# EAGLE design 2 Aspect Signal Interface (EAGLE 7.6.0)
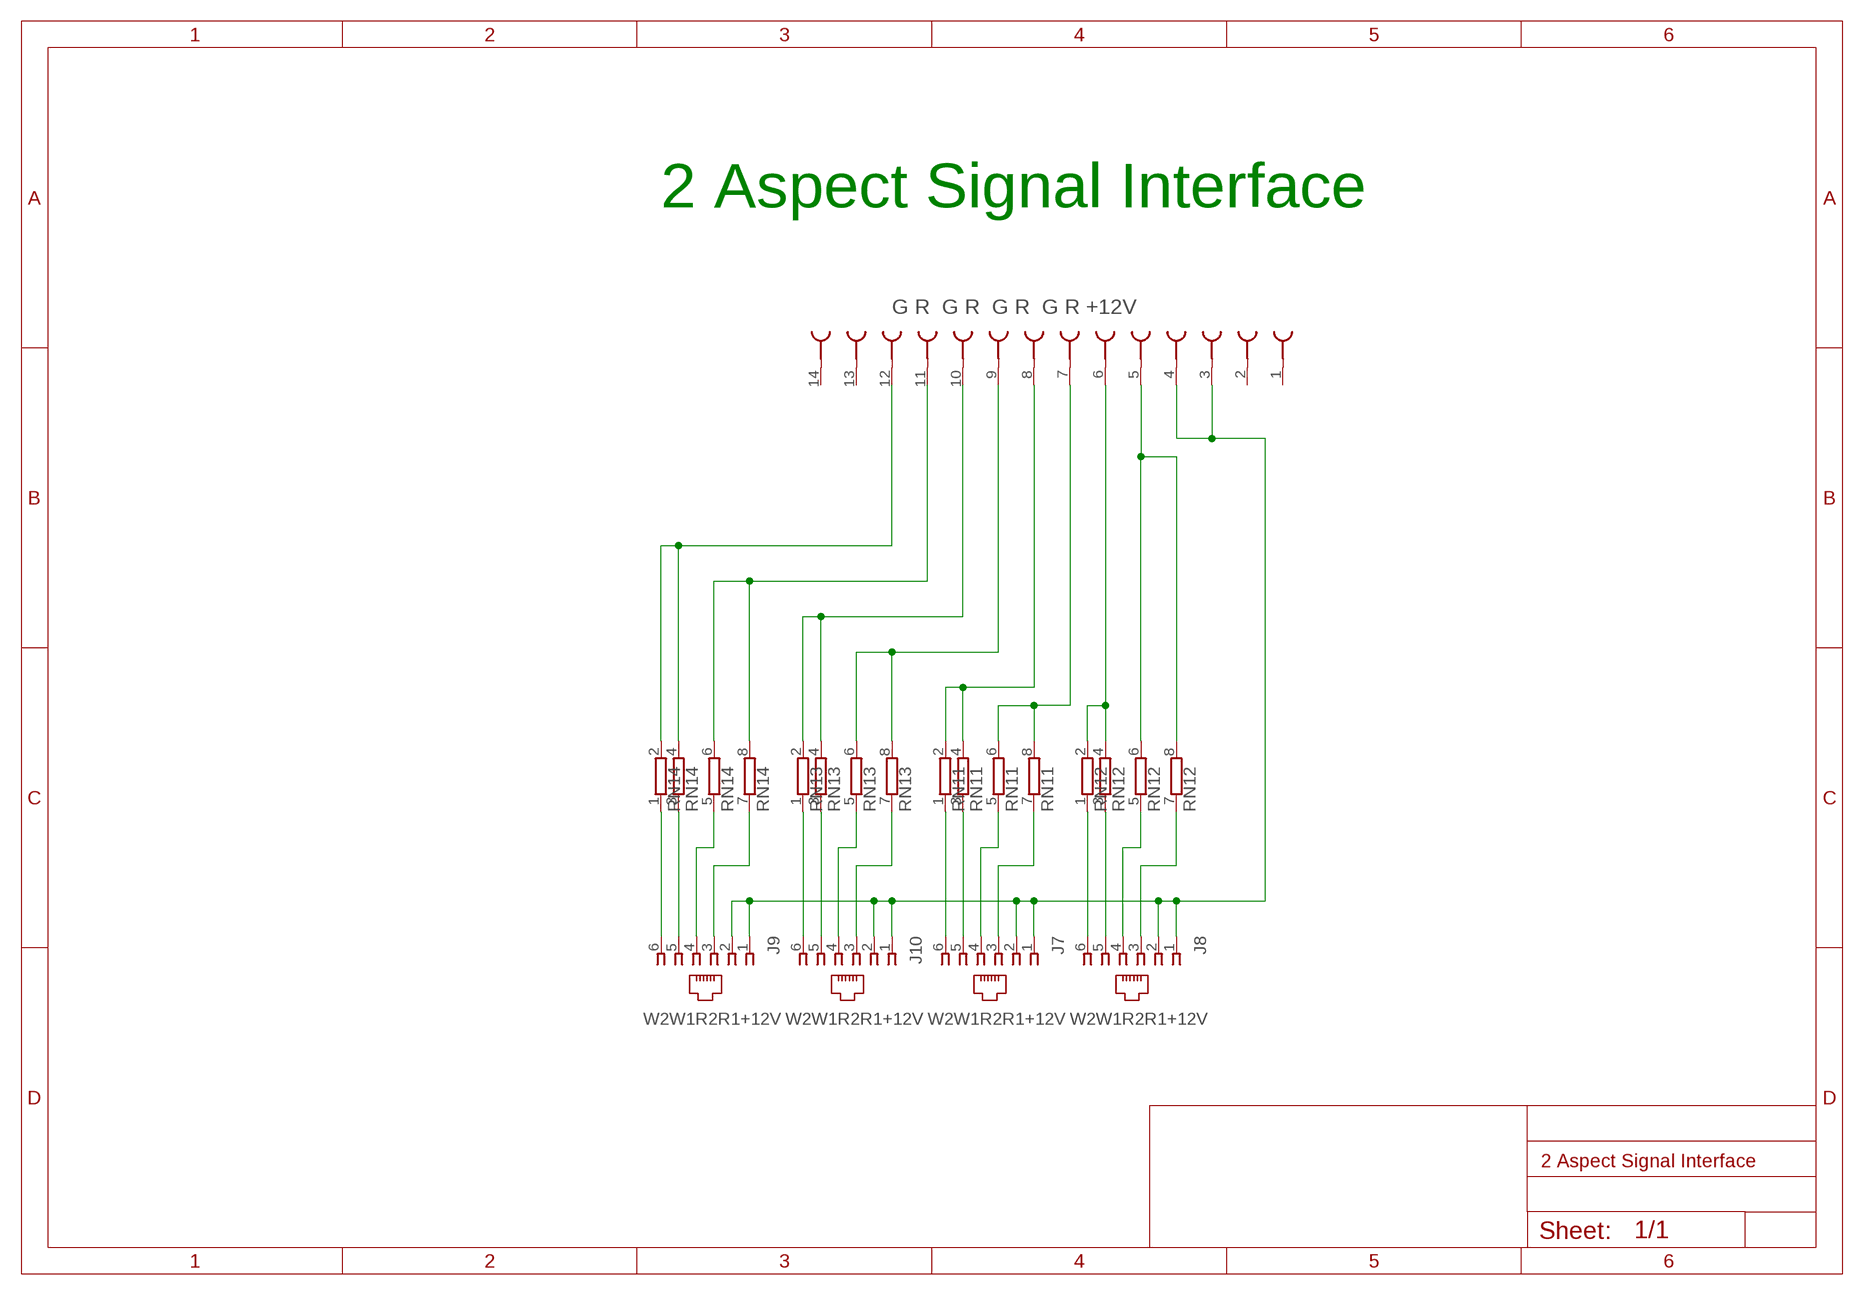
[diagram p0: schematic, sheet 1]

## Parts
J7  520250-3  [520250-3]
J8  520250-3  [520250-3]
J9  520250-3  [520250-3]
J10  520250-3  [520250-3]
RN11  E4RP  [SIL8]
RN12  E4RP  [SIL8]
RN13  E4RP  [SIL8]
RN14  E4RP  [SIL8]
U$16  AMP_FEMALE_PLUG  [AMP_FEMALE_PLUG]

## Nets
N$65: RN12.2 RN12.4 U$16.6(SK5)
N$66: J7.4 RN11.5
N$67: J7.5 RN11.3
N$68: J7.6 RN11.1
N$69: J7.3 RN11.7
N$70: J10.4 RN13.5
N$71: J8.5 RN12.3
N$72: J8.6 RN12.1
N$73: RN12.6 RN12.8 U$16.5(SK4)
N$74: J8.4 RN12.5
N$75: J10.3 RN13.7
N$76: RN11.6 RN11.8 U$16.7(SK6)
N$77: J8.3 RN12.7
N$78: J10.5 RN13.3
N$79: J10.6 RN13.1
N$80: J9.4 RN14.5
N$81: J9.3 RN14.7
N$85: J9.5 RN14.3
N$86: J9.6 RN14.1
N$87: J7.1 J7.2 J8.1 J8.2 J9.1 J9.2 J10.1 J10.2 U$16.3(SK2) U$16.4(SK3)
N$89: RN11.2 RN11.4 U$16.8(SK7)
N$90: RN13.6 RN13.8 U$16.9(SK8)
N$91: RN13.2 RN13.4 U$16.10(SK9)
N$92: RN14.6 RN14.8 U$16.11(SK10)
N$93: RN14.2 RN14.4 U$16.12(SK11)
Unconnected: U$16.1(SK) U$16.2(SK1) U$16.13(SK12) U$16.14(SK13)

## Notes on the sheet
- 2 Aspect Signal Interface
- G R  G R  G R  G R +12V
- W2W1R2R1+12V | W2W1R2R1+12V | W2W1R2R1+12V | W2W1R2R1+12V

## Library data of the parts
J7-J10 = con-amp:520250-3: AMP connector; MF: TYCO ELECTRONICS; MPN: 5520250-3; OC_FARNELL: unknown; OC_NEWARK: 42K8724
RN11-RN14 = resistor-sil:E4RP: SIL RESISTOR; OC_FARNELL: unknown; OC_NEWARK: unknown
U$16 = con-3m:AMP_FEMALE_PLUG

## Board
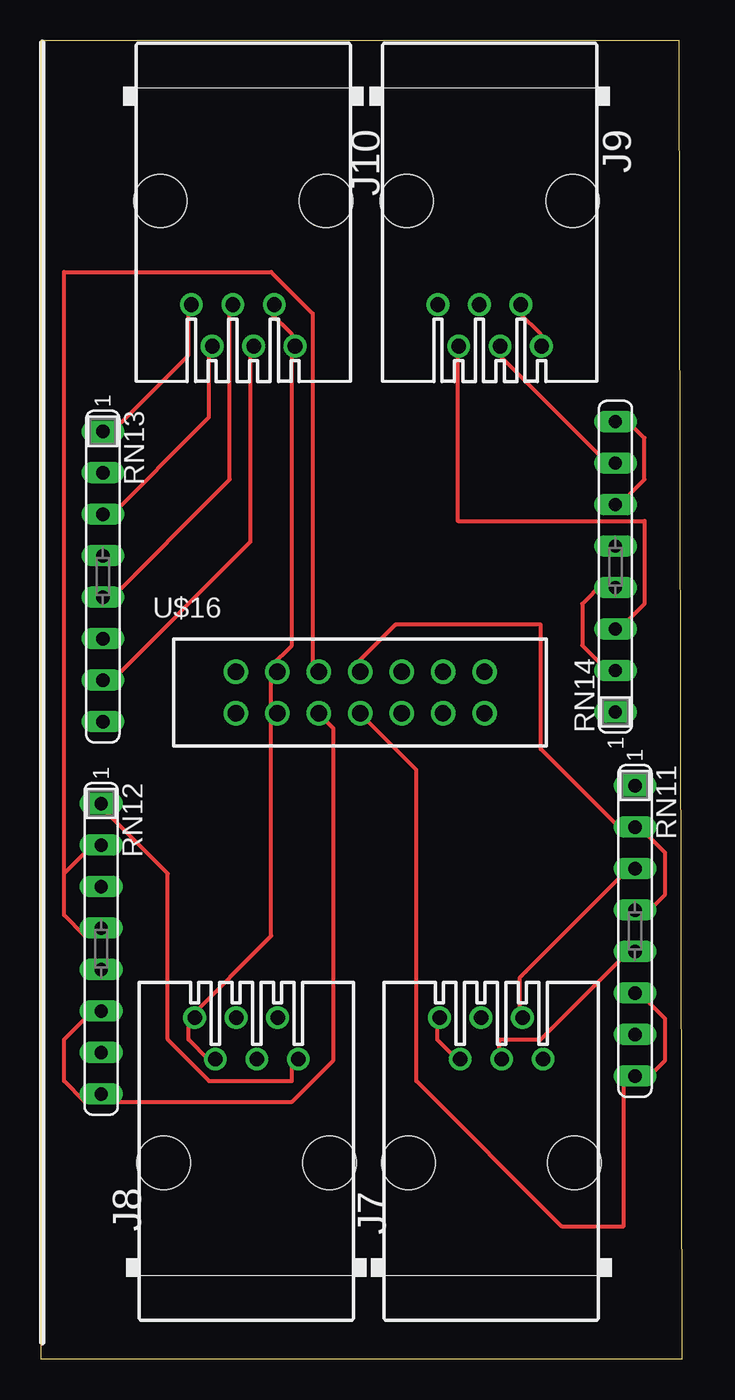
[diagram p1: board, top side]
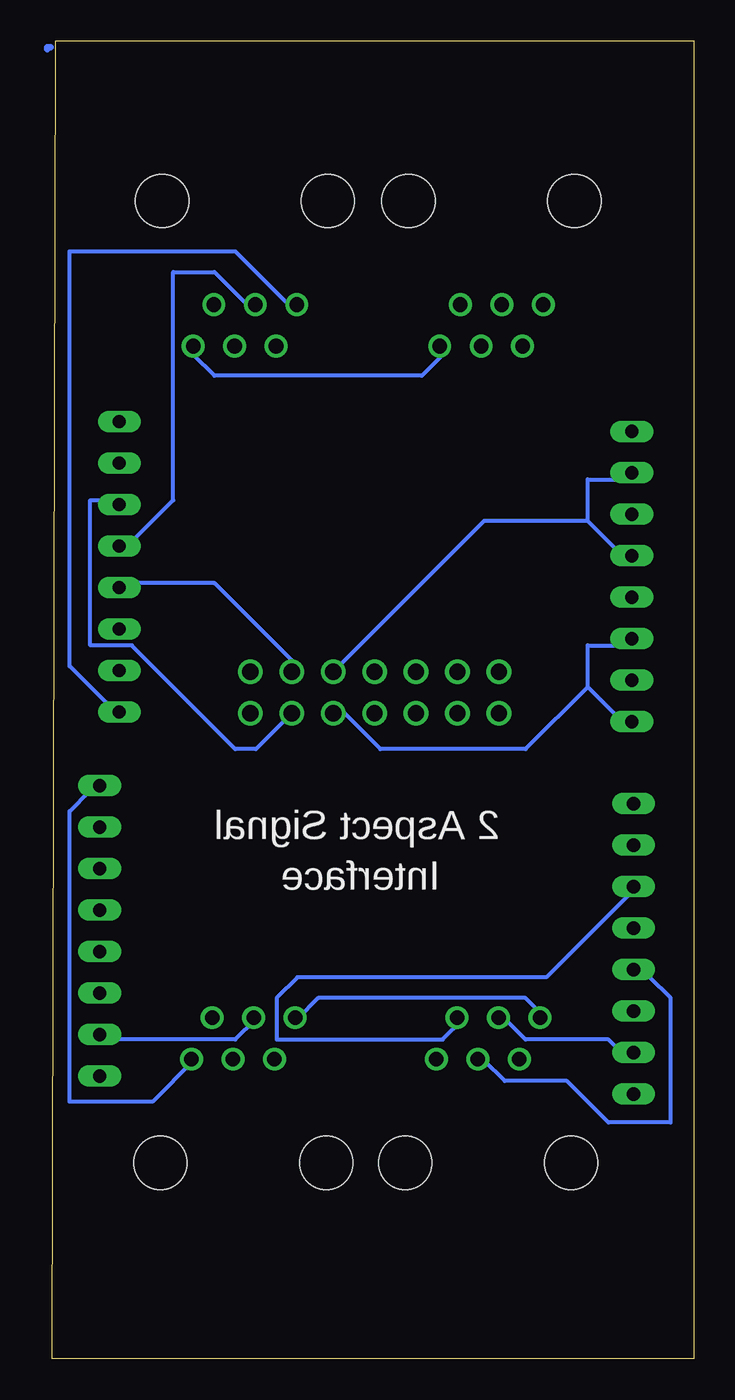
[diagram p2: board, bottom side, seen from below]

Size 39.3 x 80.7 mm. Coordinates in mm from the lower left corner, seen from the top.
Outline: 0,0 39.3,0 39.1,80.7 0,80.7 0,0
Copper layers (1*16): Top 0.035mm / dielectric 1.5mm / Bottom 0.035mm
Design rules "default": minimum track width 10mil, minimum drill 24mil, track to track 8mil, track to pad 8mil, pad to pad 8mil, via to via 8mil, smd to smd 8mil, copper to edge 40mil, drill to drill 8mil, minimum pad ring 10mil, minimum via ring 8mil, stop-mask expansion 4mil, vias tented up to drill 0mil, thermal gap 10mil

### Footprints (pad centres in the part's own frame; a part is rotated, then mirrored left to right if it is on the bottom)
520250-3 = drill 0.889: 1 -3.175,8.89; 2 -1.905,6.35; 3 -0.635,8.89; 4 0.635,6.35; 5 1.905,8.89; 6 3.175,6.35 | hole 3.251: -5.08,0; 5.08,0
SIL8 = drill 0.813 long: 1 -8.89,0; 2 -6.35,0; 3 -3.81,0; 4 -1.27,0; 5 1.27,0; 6 3.81,0; 7 6.35,0; 8 8.89,0
AMP_FEMALE_PLUG = drill 1 pad 1.422: 1 -10.16,-1.27; 2 -10.16,1.27; 3 -7.62,-1.27; 4 -7.62,1.27; 5 -5.08,-1.27; 6 -5.08,1.27; 7 -2.54,-1.27; 8 -2.54,1.27; 9 0,-1.27; 10 0,1.27; 11 2.54,-1.27; 12 2.54,1.27; 13 5.08,-1.27; 14 5.08,1.27

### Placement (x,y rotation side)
J7  27.6,12 0 top
J8  12.6,12 0 top
J9  27.5,70.9 180 top
J10  12.4,70.9 180 top
RN11  36.4,26.2 270 top
RN12  3.7,25.1 270 top
RN13  3.8,47.9 270 top
RN14  35.2,48.5 90 top
U$16  22.1,40.8 0 top

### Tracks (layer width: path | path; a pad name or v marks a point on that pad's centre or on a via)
N$65
  Top 0.254: 1.42,29.71 1.42,27.17 2.69,25.9 RN12.4 | 1.42,29.71 2.69,30.98 RN12.2 | 1.42,29.71 1.42,66.54 14.12,66.54 16.66,64 16.66,42.41 U$16.6
N$66
  Top 0.254: RN11.5 35.71,24.63 30.63,19.55 28.09,19.55 28.09,18.28 J7.4
N$67
  Top 0.254: RN11.3 35.71,29.71 29.36,23.36 29.36,20.82 J7.5
N$68
  Bottom 0.254: RN11.1 36.98,34.79 38.25,33.52 38.25,15.74 33.17,15.74 30.63,18.28 J7.6
N$69
  Bottom 0.254: RN11.7 35.71,19.55 28.09,19.55 26.82,20.82 J7.3
N$70
  Top 0.254: RN13.5 3.96,46.22 11.58,53.84 11.58,64 J10.4
N$71
  Bottom 0.254: RN12.3 3.96,28.44 9.04,23.36 24.28,23.36 25.55,22.09 25.55,19.55 15.39,19.55 14.12,20.82 J8.5
N$72
  Top 0.254: RN12.1 3.96,33.52 7.77,29.71 7.77,19.55 10.31,17.01 15.39,17.01 15.39,18.28 J8.6
N$73
  Top 0.254: RN12.6 2.69,20.82 1.42,19.55 1.42,17.01 2.69,15.74 RN12.8 3.96,15.74 15.39,15.74 17.93,18.28 17.93,38.6 16.66,39.87 U$16.5
N$74
  Bottom 0.254: RN12.5 2.69,23.36 1.42,22.09 1.42,14.47 5.23,14.47 7.77,17.01 11.58,17.01 12.85,18.28 J8.4
N$75
  Top 0.254: RN13.7 3.96,41.14 12.85,50.03 12.85,61.46 J10.3
N$76
  Top 0.254: RN11.6 36.98,22.09 38.25,20.82 38.25,18.28 36.98,17.01 RN11.8 35.71,17.01 35.71,8.12 31.9,8.12 23.01,17.01 23.01,36.06 19.2,39.87 U$16.7
N$77
  Bottom 0.254: RN12.7 3.96,18.28 5.23,19.55 10.31,19.55 11.58,20.82 J8.3
N$78
  Top 0.254: RN13.3 3.96,51.3 10.31,57.65 10.31,61.46 J10.5
N$79
  Top 0.254: RN13.1 3.96,56.38 9.04,61.46 9.04,64 J10.6
N$80
  Bottom 0.254: RN14.5 34.44,50.03 31.9,52.57 31.9,66.54 29.36,66.54 26.82,64 J9.4
N$81
  Top 0.254: RN14.7 34.44,55.11 28.09,61.46 J9.3
N$83
  Bottom 0.406: 39.4,80.3 39.6,80.3 39.6,80.2
N$85
  Top 0.254: RN14.3 35.71,44.95 36.98,46.22 36.98,51.3 25.55,51.3 25.55,61.46 J9.5
N$86
  Bottom 0.254: RN14.1 35.71,39.87 38.25,42.41 38.25,67.81 28.09,67.81 24.28,64 J9.6
N$87
  Top 0.254: J9.2 29.36,64 30.63,62.73 30.63,61.46 J9.1 | J7.2 25.55,18.28 24.28,19.55 24.28,20.82 J7.1 | 9.04,20.82 9.04,19.55 10.31,18.28 J8.2 | 14.12,39.87 14.12,42.41 | 15.39,61.46 15.39,62.73 14.12,64 J10.2 | 14.12,42.41 15.39,43.68 15.39,61.46 | 14.12,42.41 U$16.4 | 15.39,61.46 J10.1 | 9.04,20.82 14.12,25.9 14.12,39.87 | 9.04,20.82 J8.1 | 14.12,39.87 U$16.3
  Bottom 0.254: J7.1 24.28,20.82 23.01,22.09 10.31,22.09 9.04,20.82 J8.1 | J9.1 30.63,61.46 29.36,60.19 16.66,60.19 15.39,61.46 J10.1
N$89
  Top 0.254: RN11.4 36.98,27.17 38.25,28.44 38.25,30.98 36.98,32.25 RN11.2 35.71,32.25 30.63,37.33 30.63,44.95 21.74,44.95 19.2,42.41 U$16.8
N$90
  Bottom 0.254: 6.5,41.14 3.96,38.6 RN13.8 | 6.5,41.14 6.5,43.68 3.96,43.68 RN13.6 | 6.5,41.14 10.31,37.33 19.2,37.33 21.74,39.87 U$16.9
N$91
  Bottom 0.254: 6.5,51.3 3.96,48.76 RN13.4 | 6.5,51.3 6.5,53.84 3.96,53.84 RN13.2 | 6.5,51.3 12.85,51.3 21.74,42.41 U$16.10
N$92
  Top 0.254: RN14.6 35.71,52.57 36.98,53.84 36.98,56.38 35.71,57.65 RN14.8
  Bottom 0.254: U$16.11 24.28,39.87 26.82,37.33 28.09,37.33 34.44,43.68 36.98,43.68 36.98,52.57 35.71,52.57 RN14.6
N$93
  Top 0.254: RN14.2 34.44,42.41 33.17,43.68 33.17,46.22 34.44,47.49 RN14.4
  Bottom 0.254: U$16.12 24.28,42.41 29.36,47.49 34.44,47.49 RN14.4

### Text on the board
bPlace: 2 Aspect Signal | Interface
